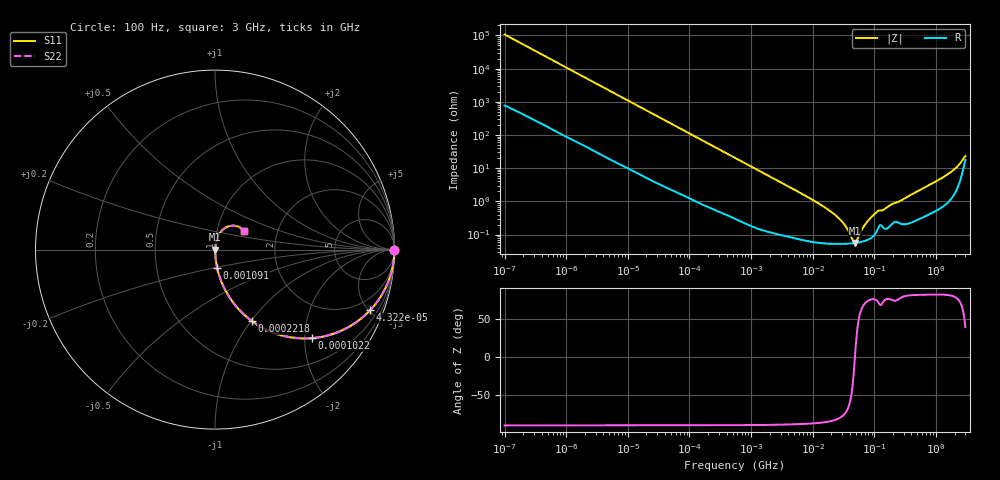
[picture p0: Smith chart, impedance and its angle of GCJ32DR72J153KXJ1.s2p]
!Murata Part Number: GCJ32DR72J153KXJ1
!These Parameters are Measured in Series Mode Connection
!Data Generated on Mar 13, 2026
!  o--ll--o
!Port1  Port2
!  o------o
!Operation Temp=25[degC], DC Bias Voltage=0[V]
!Freq. Start=100[Hz] Stop=3[GHz] 401[Steps]
# Hz S RI R 50
!Freq.(Hz) S11(Real) S11(Imag) S21(Real) S21(Imag) S12(Real) S12(Imag) S22(Real) S22(Imag)
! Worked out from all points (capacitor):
!   401 points, 100 Hz to 3 GHz, reference 50 ohm
!   read as one part in series: C = 14.9 nF near 109 Hz
!   lowest |Z| = 55.8 mohm at 48.15 MHz (marker M1)
!   series resonance near 48.35 MHz, so ESL is about 730 pH
!   S11 on the Smith chart (normalised r, x): 100 Hz: open; 43.22 kHz: 1.05, -5.11; 102.2 kHz: 1.02, -2.17; 221.8 kHz: 1.01, -1.01; 1.091 MHz: 1.00, -0.21; 3 GHz: 1.36, +0.30
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100  1 -0.000936  7.6e-06 0.000936  7.6e-06 0.000936  1 -0.000936
1788  0.9996 -0.0165  0.000412 0.0165  0.000412 0.0165  0.9996 -0.0165
9582  0.9916 -0.0867  0.00837 0.0867  0.00837 0.0867  0.9916 -0.0867
31977  0.9202 -0.2662  0.0798 0.2662  0.0798 0.2662  0.9202 -0.2662
43220  0.8646 -0.3372  0.1354 0.3372  0.1354 0.3372  0.8646 -0.3372
102221  0.5409 -0.4928  0.4591 0.4928  0.4591 0.4928  0.5409 -0.4928
221826  0.2049 -0.3976  0.7951 0.3976  0.7951 0.3976  0.2049 -0.3976
547723  0.0431 -0.1959  0.9569 0.1959  0.9569 0.1959  0.0431 -0.1959
1090550  0.0123 -0.1022  0.9878 0.1022  0.9878 0.1022  0.0123 -0.1022
9794414  0.000724 -0.0113  0.9993 0.0113  0.9993 0.0113  0.000724 -0.0113
2.635803e7  0.000531 -0.00309  0.9995 0.00309  0.9995 0.00309  0.000531 -0.00309
3.412477e7  0.000531 -0.0017  0.9995 0.0017  0.9995 0.0017  0.000531 -0.0017
4.418008e7  0.000547 -0.000434  0.9995 0.000434  0.9995 0.000434  0.000547 -0.000434
4.815176e7  0.000557 -1.91e-05  0.9994 1.91e-05  0.9994 1.91e-05  0.000557 -1.91e-05
5.248048e7  0.00057 0.000397  0.9994 -0.000397  0.9994 -0.000397  0.00057 0.000397
7.093284e7  0.000652 0.00192  0.9993 -0.00192  0.9993 -0.00192  0.000652 0.00192
9.183415e7  0.000839 0.00342  0.9992 -0.00342  0.9992 -0.00342  0.000839 0.00342
1.138854e8  0.0015 0.00487  0.9985 -0.00487  0.9985 -0.00487  0.0015 0.00487
1.751444e8  0.00177 0.00724  0.9982 -0.00724  0.9982 -0.00724  0.00177 0.00724
1.324213e9  0.00994 0.053  0.9901 -0.053  0.9901 -0.053  0.00994 0.053
2.219584e9  0.0351 0.1028  0.9649 -0.1028  0.9649 -0.1028  0.0351 0.1028
3e9  0.1642 0.1049  0.8358 -0.1049  0.8358 -0.1049  0.1642 0.1049
